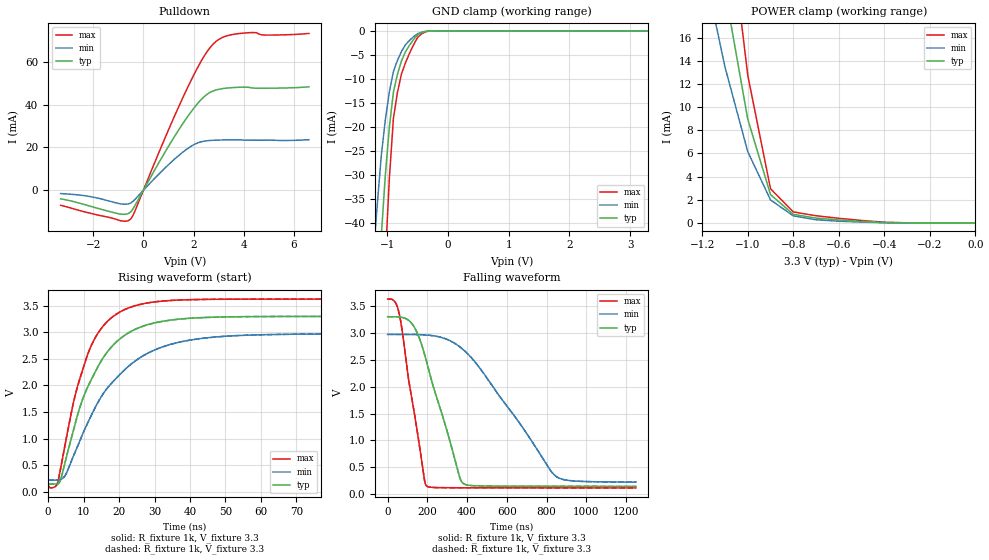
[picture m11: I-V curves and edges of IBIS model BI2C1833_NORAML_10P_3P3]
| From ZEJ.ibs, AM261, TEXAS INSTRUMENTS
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[Model]   BI2C1833_NORAML_10P_3P3
Model_type   I/O_open_drain
Polarity   Non-Inverting
Enable   Active-Low
Vinl =  0.99
Vinh =  2.31
Cref =  400pF
Rref =  528
Vref =  1.8V
Vmeas =  1.65
C_comp   3.826936p   2.767369p   5.268171p
|[Input load] normal
|[Output drive] i2c standard
|[supplytol] 10
|[temp] ind
[Model Spec]
Vinl   0.99   0.891   1.089
Vinh   2.31   2.079   2.541
[Temperature Range]   25   125   -40
[Voltage Range]   3.3   2.97   3.63
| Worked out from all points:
|   slope of the pulldown table from 0 to 0.495 V, typ, clamps not added: 47.7 ohm
|   GND clamp passes 1 mA (typ) near -0.51 V on its own axis
|   POWER clamp passes 1 mA (typ) near -0.81 V on its own axis
|   rising waveform, R_fixture 1k, V_fixture 3.3: 20-80 % time 11.5ns typ, 16ns min, 8.93ns max; typ from 0.148 V to 3.29 V
|   rising waveform, R_fixture 1k, V_fixture 3.3: 20-80 % time 11.5ns typ, 16ns min, 8.93ns max; typ from 0.148 V to 3.29 V
|   falling waveform, R_fixture 1k, V_fixture 3.3: 20-80 % time 149ns typ, 315ns min, 85.8ns max; typ from 3.29 V to 0.148 V
|   falling waveform, R_fixture 1k, V_fixture 3.3: 20-80 % time 149ns typ, 315ns min, 85.8ns max; typ from 3.29 V to 0.148 V
| Nom Voltages:
|   VDD=1.1001, VDDS=3.3, VDDS18=1.8, ESD_BIASFET=0, VSS=0, VSSS=0
| Min Voltages:
|   VDD=0.99, VDDS=2.97, VDDS18=1.62, ESD_BIASFET=0, VSS=0, VSSS=0
| Max Voltages:
|   VDD=1.21, VDDS=3.63, VDDS18=1.98, ESD_BIASFET=0, VSS=0, VSSS=0
[POWER_clamp]
|   voltage   I(typ)   I(min)   I(max)
-3.3V     371.9mA    370.7mA    506.1mA
-1.133V   24.49mA    16.53mA    35.37mA
-1.1V     20.05mA    13.45mA    29.08mA
-1.067V   16.35mA    11.02mA    23.63mA
-1.033V   12.65mA    8.589mA    18.19mA
-1V       8.957mA    6.157mA    12.75mA
-900mV    2.454mA    1.995mA    2.958mA
-800mV    749.9uA    620.3uA    962.7uA
-700mV    426.8uA    282.9uA    630.6uA
-400mV    48.77uA    29.05uA    73.94uA
0V        4.596uA    2.036uA    9.305uA
[Pulldown]
|   voltage   I(typ)   I(min)   I(max)
-3.3V     -3.962mA   -1.526mA   -6.996mA
-2.1V     -7.46mA    -2.966mA   -10.74mA
-1V       -10.91mA   -6.109mA   -13.87mA
-600mV    -10.84mA   -6.367mA   -14.18mA
-400mV    -8.438mA   -5.006mA   -11.41mA
800mV     16.55mA    9.687mA    22.68mA
1.7V      33.31mA    18.95mA    46.4mA
2.3V      42.31mA    22.63mA    60.18mA
2.8V      46.45mA    23.36mA    68.46mA
3.2V      47.54mA    23.51mA    71.56mA
3.9V      48.12mA    23.53mA    73.26mA
6.6V      48.3mA     23.61mA    73.21mA
[GND_clamp]
|   voltage   I(typ)   I(min)   I(max)
-3.3V     -732.9mA   -579.5mA   -1.135A
-1.233V   -77.75mA   -47.44mA   -124.9mA
-1.167V   -59.87mA   -36.39mA   -96.3mA
-1.1V     -42.93mA   -26.1mA    -68.88mA
-1.033V   -30.16mA   -18.6mA    -47.71mA
-966.7mV  -20.1mA    -12.73mA   -30.84mA
-900mV    -12.77mA   -8.484mA   -18.26mA
-833.3mV  -9.047mA   -6.154mA   -12.83mA
-700mV    -4.35mA    -2.882mA   -6.627mA
-500mV    -792.1uA   -572.8uA   -1.328mA
-300mV    -20.03uA   -28.11uA   -28.26uA
3.3V      4.596uA    11.21uA    5.613uA
[Ramp]
| variable   typ   min   max
dV/dt_f  1.8954887/0.1492067u  1.6524661/0.31643332u  2.1103219/86.143627n
dV/dt_r 85.087907m/13.236053n  77.98547m/6.4033251n 80.131523m/8.972681n
R_load = 1k
[Rising Waveform]
R_fixture = 1k
V_fixture = 3.3
V_fixture_min = 2.97
V_fixture_max = 3.63
|   time   V(typ)   V(min)   V(max)
0s        148.1mV    220.5mV    120.2mV
2.643ns   148.1mV    220.5mV    164.3mV
4.908ns   592mV      319.4mV    942.1mV
8.168ns   1.419V     836.1mV    1.954V
11.44ns   2.011V     1.337V     2.635V
14.54ns   2.414V     1.74V      3.031V
23.16ns   3.008V     2.388V     3.469V
36.72ns   3.245V     2.809V     3.604V
79.13ns   3.297V     2.967V     3.622V
1.25us    3.295V     2.968V     3.621V
[Rising Waveform]
R_fixture = 1k
V_fixture = 3.3
V_fixture_min = 2.97
V_fixture_max = 3.63
|   time   V(typ)   V(min)   V(max)
0s        148.1mV    220.5mV    120.2mV
2.643ns   148.1mV    220.5mV    164.3mV
4.908ns   592mV      319.4mV    942.1mV
8.168ns   1.419V     836.1mV    1.954V
11.44ns   2.011V     1.337V     2.635V
14.54ns   2.414V     1.74V      3.031V
23.16ns   3.008V     2.388V     3.469V
36.72ns   3.245V     2.809V     3.604V
79.13ns   3.297V     2.967V     3.622V
1.25us    3.295V     2.968V     3.621V
[Falling Waveform]
R_fixture = 1k
V_fixture = 3.3
V_fixture_min = 2.97
V_fixture_max = 3.63
|   time   V(typ)   V(min)   V(max)
0s        3.295V     2.967V     3.621V
37.3ns    3.295V     2.967V     3.569V
62.07ns   3.29V      2.967V     3.287V
131.5ns   3.119V     2.966V     1.575V
185.2ns   2.609V     2.959V     272.9mV
196.8ns   2.454V     2.956V     155mV
361ns     339.1mV    2.743V     122.6mV
383.3ns   195.8mV    2.676V     122.4mV
844ns     149.5mV    344.8mV    121.2mV
1.25us    148.5mV    227.9mV    121.1mV
[Falling Waveform]
R_fixture = 1k
V_fixture = 3.3
V_fixture_min = 2.97
V_fixture_max = 3.63
|   time   V(typ)   V(min)   V(max)
0s        3.295V     2.967V     3.621V
37.3ns    3.295V     2.967V     3.569V
62.07ns   3.29V      2.967V     3.287V
131.5ns   3.119V     2.966V     1.575V
185.2ns   2.609V     2.959V     272.9mV
196.8ns   2.454V     2.956V     155mV
361ns     339.1mV    2.743V     122.6mV
383.3ns   195.8mV    2.676V     122.4mV
844ns     149.5mV    344.8mV    121.2mV
1.25us    148.5mV    227.9mV    121.1mV
